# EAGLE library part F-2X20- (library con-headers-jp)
FEMALE HEADER
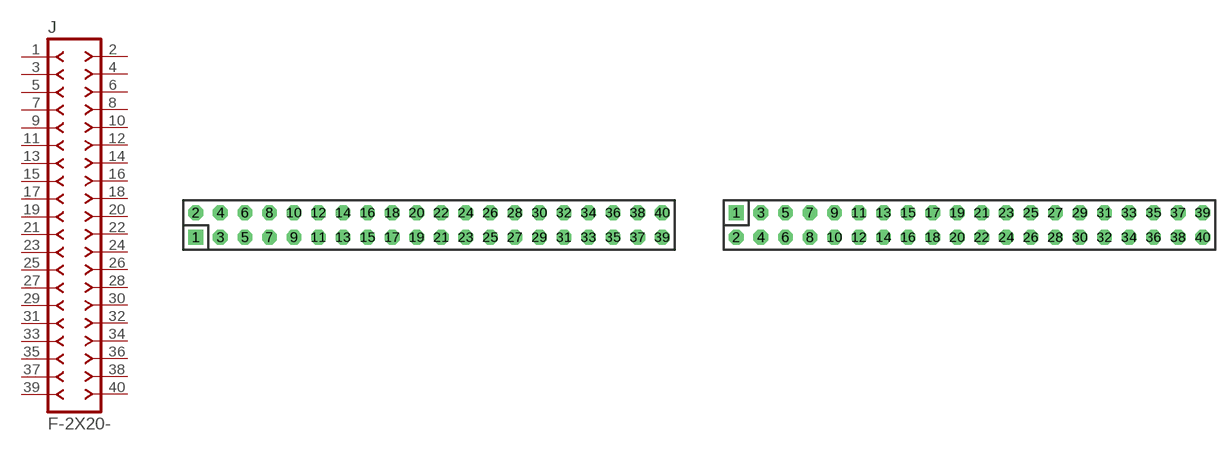
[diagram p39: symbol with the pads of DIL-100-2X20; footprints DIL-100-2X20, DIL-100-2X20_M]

Designator prefix J

## F-2X20-DIL-100  [DIL-100-2X20]
1  1  pas
2  2  pas
3  3  pas
4  4  pas
5  5  pas
6  6  pas
7  7  pas
8  8  pas
9  9  pas
10  10  pas
11  11  pas
12  12  pas
13  13  pas
14  14  pas
15  15  pas
16  16  pas
17  17  pas
18  18  pas
19  19  pas
20  20  pas
21  21  pas
22  22  pas
23  23  pas
24  24  pas
25  25  pas
26  26  pas
27  27  pas
28  28  pas
29  29  pas
30  30  pas
31  31  pas
32  32  pas
33  33  pas
34  34  pas
35  35  pas
36  36  pas
37  37  pas
38  38  pas
39  39  pas
40  40  pas

## F-2X20-DIL-100_M  [DIL-100-2X20_M]
Pads as for DIL-100-2X20

## F-2X20-DIL-2MM  [DIL-2MM-2X20]
Pads as for DIL-100-2X20

## F-2X20-DIL-2MM_M  [DIL-2MM-2X20_M]
Pads as for DIL-100-2X20

## F-2X20-71991  [71991-40]
Pads as for DIL-100-2X20

## Footprint DIL-100-2X20 (pad centres in mm)
PIN HEADER - 0.1"
drill 1.016 square: 1 -24.13,-1.27
drill 1.016 octagon: 2 -24.13,1.27; 3 -21.59,-1.27; 4 -21.59,1.27; 5 -19.05,-1.27; 6 -19.05,1.27; 7 -16.51,-1.27; 8 -16.51,1.27; 9 -13.97,-1.27; 10 -13.97,1.27; 11 -11.43,-1.27; 12 -11.43,1.27; 13 -8.89,-1.27; 14 -8.89,1.27; 15 -6.35,-1.27; 16 -6.35,1.27; 17 -3.81,-1.27; 18 -3.81,1.27; 19 -1.27,-1.27; 20 -1.27,1.27; 21 1.27,-1.27; 22 1.27,1.27; 23 3.81,-1.27; 24 3.81,1.27; 25 6.35,-1.27; 26 6.35,1.27; 27 8.89,-1.27; 28 8.89,1.27; 29 11.43,-1.27; 30 11.43,1.27; 31 13.97,-1.27; 32 13.97,1.27; 33 16.51,-1.27; 34 16.51,1.27; 35 19.05,-1.27; 36 19.05,1.27; 37 21.59,-1.27; 38 21.59,1.27; 39 24.13,-1.27; 40 24.13,1.27

## Footprint DIL-100-2X20_M (pad centres in mm)
PIN HEADER - MIRRORED 0.1"
drill 1.016 square: 1 -24.13,1.27
drill 1.016 octagon: 2 -24.13,-1.27; 3 -21.59,1.27; 4 -21.59,-1.27; 5 -19.05,1.27; 6 -19.05,-1.27; 7 -16.51,1.27; 8 -16.51,-1.27; 9 -13.97,1.27; 10 -13.97,-1.27; 11 -11.43,1.27; 12 -11.43,-1.27; 13 -8.89,1.27; 14 -8.89,-1.27; 15 -6.35,1.27; 16 -6.35,-1.27; 17 -3.81,1.27; 18 -3.81,-1.27; 19 -1.27,1.27; 20 -1.27,-1.27; 21 1.27,1.27; 22 1.27,-1.27; 23 3.81,1.27; 24 3.81,-1.27; 25 6.35,1.27; 26 6.35,-1.27; 27 8.89,1.27; 28 8.89,-1.27; 29 11.43,1.27; 30 11.43,-1.27; 31 13.97,1.27; 32 13.97,-1.27; 33 16.51,1.27; 34 16.51,-1.27; 35 19.05,1.27; 36 19.05,-1.27; 37 21.59,1.27; 38 21.59,-1.27; 39 24.13,1.27; 40 24.13,-1.27

## Footprint DIL-2MM-2X20 (pad centres in mm)
PIN HEADER - 2MM
drill 0.711 square: 1 -19,-1
drill 0.711: 2 -19,1; 3 -17,-1; 4 -17,1; 5 -15,-1; 6 -15,1; 7 -13,-1; 8 -13,1; 9 -11,-1; 10 -11,1; 11 -9,-1; 12 -9,1; 13 -7,-1; 14 -7,1; 15 -5,-1; 16 -5,1; 17 -3,-1; 18 -3,1; 19 -1,-1; 20 -1,1; 21 1,-1; 22 1,1; 23 3,-1; 24 3,1; 25 5,-1; 26 5,1; 27 7,-1; 28 7,1; 29 9,-1; 30 9,1; 31 11,-1; 32 11,1; 33 13,1; 34 13,-1; 35 15,1; 36 15,-1; 37 17,1; 38 17,-1; 39 19,1; 40 19,-1

## Footprint DIL-2MM-2X20_M (pad centres in mm)
PIN HEADER - MIRRORED 2MM
drill 0.711 square: 1 -19,1
drill 0.711: 2 -19,-1; 3 -17,1; 4 -17,-1; 5 -15,1; 6 -15,-1; 7 -13,1; 8 -13,-1; 9 -11,1; 10 -11,-1; 11 -9,1; 12 -9,-1; 13 -7,1; 14 -7,-1; 15 -5,1; 16 -5,-1; 17 -3,1; 18 -3,-1; 19 -1,1; 20 -1,-1; 21 1,1; 22 1,-1; 23 3,1; 24 3,-1; 25 5,1; 26 5,-1; 27 7,1; 28 7,-1; 29 9,1; 30 9,-1; 31 11,1; 32 11,-1; 33 13,-1; 34 13,1; 35 15,-1; 36 15,1; 37 17,-1; 38 17,1; 39 19,-1; 40 19,1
